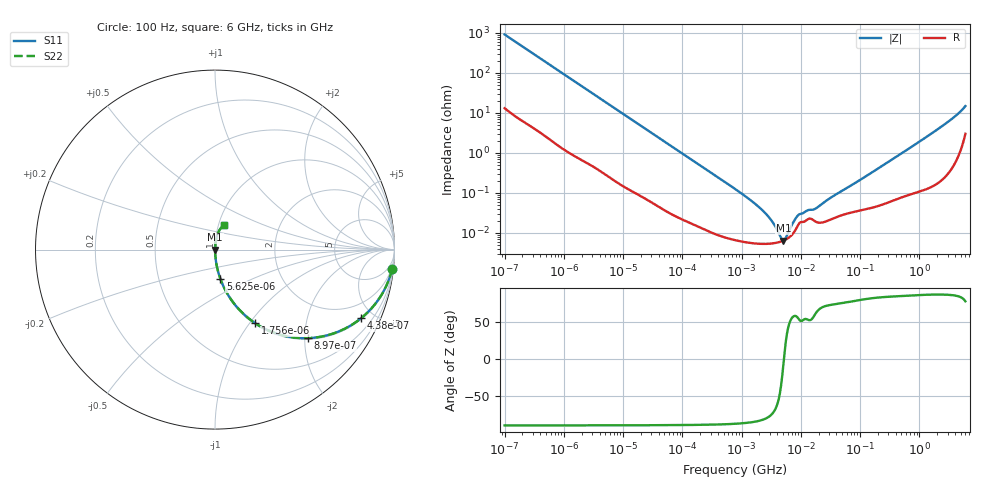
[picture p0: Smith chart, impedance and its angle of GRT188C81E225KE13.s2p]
!Murata Part Number: GRT188C81E225KE13
!These Parameters are Measured in Series Mode Connection
!Data Generated on Jun 19, 2026
!  o--ll--o
!Port1  Port2
!  o------o
!Operation Temp=25[degC], DC Bias Voltage=0[V]
!Freq. Start=100[Hz] Stop=6[GHz] 401[Steps]
# Hz S RI R 50
!Freq.(Hz) S11(Real) S11(Imag) S21(Real) S21(Imag) S12(Real) S12(Imag) S22(Real) S22(Imag)
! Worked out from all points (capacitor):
!   401 points, 100 Hz to 6 GHz, reference 50 ohm
!   read as one part in series: C = 1.74 uF near 109 Hz
!   lowest |Z| = 6.44 mohm at 5.079 MHz (marker M1)
!   series resonance near 5.176 MHz, so ESL is about 540 pH
!   S11 on the Smith chart (normalised r, x): 100 Hz: 1, -18; 438 Hz: 1.06, -4.22; 897 Hz: 1.03, -2.07; 1.756 kHz: 1.01, -1.06; 5.625 kHz: 1.01, -0.34; 6 GHz: 1.06, +0.29
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100  0.9867 -0.1078  0.0133 0.1078  0.0133 0.1078  0.9867 -0.1078
245  0.9309 -0.2469  0.0691 0.2469  0.0691 0.2469  0.9309 -0.2469
438  0.8133 -0.3828  0.1867 0.3828  0.1867 0.3828  0.8133 -0.3828
897  0.518 -0.4932  0.482 0.4932  0.482 0.4932  0.518 -0.4932
1756  0.224 -0.4101  0.776 0.4101  0.776 0.4101  0.224 -0.4101
2008  0.1819 -0.3787  0.8181 0.3787  0.8181 0.3787  0.1819 -0.3787
3143  0.0856 -0.2723  0.9144 0.2723  0.9144 0.2723  0.0856 -0.2723
5625  0.0298 -0.1627  0.9702 0.1627  0.9702 0.1627  0.0298 -0.1627
13169  0.00635 -0.0718  0.9937 0.0718  0.9937 0.0718  0.00635 -0.0718
40335  0.00102 -0.0239  0.999 0.0239  0.999 0.0239  0.00102 -0.0239
774597  6.76e-05 -0.00126  0.9999 0.00126  0.9999 0.00126  6.76e-05 -0.00126
2074311  5.35e-05 -0.000409  0.9999 0.000409  0.9999 0.000409  5.35e-05 -0.000409
2967816  5.38e-05 -0.00023  0.9999 0.00023  0.9999 0.00023  5.38e-05 -0.00023
4246196  5.86e-05 -7.92e-05  0.9999 7.92e-05  0.9999 7.92e-05  5.86e-05 -7.92e-05
5079039  6.4e-05 -7.5e-06  0.9999 7.5e-06  0.9999 7.5e-06  6.4e-05 -7.5e-06
6075234  7.37e-05 6.57e-05  0.9999 -6.57e-05  0.9999 -6.57e-05  7.37e-05 6.57e-05
7947587  0.000112 0.000184  0.9999 -0.000184  0.9999 -0.000184  0.000112 0.000184
9090158  0.000161 0.000231  0.9998 -0.000231  0.9998 -0.000231  0.000161 0.000231
1.555665e7  0.000218 0.00031  0.9998 -0.00031  0.9998 -0.00031  0.000218 0.00031
3.124326e8  0.000629 0.00617  0.9994 -0.00617  0.9994 -0.00617  0.000629 0.00617
2.34314e9  0.00403 0.0447  0.996 -0.0447  0.996 -0.0447  0.00403 0.0447
6e9  0.0482 0.1343  0.9518 -0.1343  0.9518 -0.1343  0.0482 0.1343
